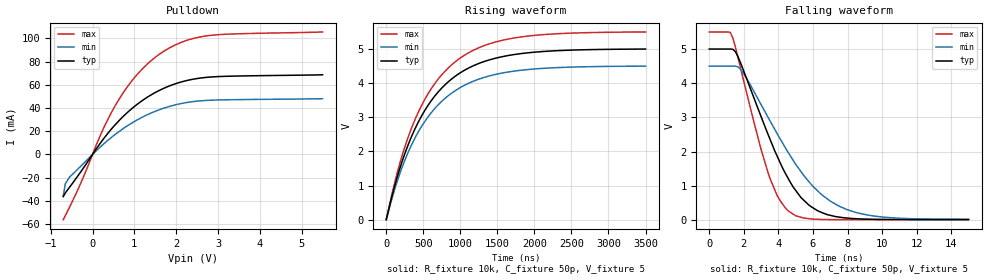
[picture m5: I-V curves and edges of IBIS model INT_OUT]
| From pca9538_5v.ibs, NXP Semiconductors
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[Model]   INT_OUT
Model_type Open_drain
Vref=5
Vmeas=2.5
Rref=10k
Cref=50p
C_comp   5.2p   5p   5.4p
[Temperature Range] 27   85   -40
[Voltage Range]   5   4.5   5.5
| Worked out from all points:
|   slope of the pulldown table from 0 to 0.75 V, typ, clamps not added: 22.5 ohm
|   falling waveform, R_fixture 10k, C_fixture 50p, V_fixture 5: 20-80 % time 2.54ns typ, 3.39ns min, 1.77ns max; typ from 5 V to 0.009 V
|   rising waveform, R_fixture 10k, C_fixture 50p, V_fixture 5: 20-80 % time 701ns typ, 702ns min, 700ns max; typ from 0.009 V to 5 V
[Pulldown]
-700mV    -36.23mA   -35.84mA   -56.1mA
-650mV    -33.03mA   -25.2mA    -52.64mA
-550mV    -28.25mA   -19.51mA   -45.37mA
-250mV    -13.34mA   -8.977mA   -22.12mA
200mV     10.42mA    6.906mA    17.51mA
550mV     25.9mA     17.48mA    42.46mA
1V        41.24mA    28.34mA    65.98mA
1.25V     47.87mA    33.16mA    75.75mA
1.55V     54.26mA    37.86mA    84.97mA
2.1V      62.18mA    43.68mA    96.14mA
2.7V      66.26mA    46.46mA    101.9mA
5.5V      68.56mA    47.97mA    105.4mA
[Falling Waveform]
R_fixture=10k
C_fixture=50p
V_fixture=5
V_fixture_min=4.5
V_fixture_max=5.5
0s        5V         4.5V       5.5V
1.212ns   5V         4.5V       5.49V
1.364ns   4.994V     4.5V       5.325V
1.97ns    4.389V     4.296V     4.116V
3.485ns   2.4V       2.926V     1.254V
3.939ns   1.853V     2.514V     702.4mV
4.545ns   1.232V     1.989V     273.9mV
5.909ns   381.7mV    1.035V     27.4mV
8.03ns    50.6mV     290mV      6.222mV
15ns      9.145mV    14.72mV    5.882mV
[Rising Waveform]
R_fixture=10k
C_fixture=50p
V_fixture=5
V_fixture_min=4.5
V_fixture_max=5.5
0s        9.123mV    12.52mV    5.881mV
106.1ns   927.8mV    835.5mV    1.021V
212.1ns   1.694V     1.524V     1.866V
318.2ns   2.318V     2.084V     2.552V
424.2ns   2.824V     2.539V     3.109V
671.7ns   3.664V     3.296V     4.034V
989.9ns   4.287V     3.857V     4.719V
1.343us   4.646V     4.18V      5.112V
1.803us   4.857V     4.371V     5.344V
3.5us     4.995V     4.495V     5.494V
[Ramp]
R_load=10k
dV/dt_r   2.494E+0/7.049E-9   2.381E+0/7.157E-9   2.616E+0/6.815E-9
dV/dt_f   2.995E+0/9.242E-11   2.992E+0/1.525E-10   2.997E+0/6.587E-11
|[End   INT_OUT
